FUNCTION "Gest Output" : VOID
TITLE =Gestione Output
AUTHOR : MassimoZ
FAMILY : NovaSrl
VERSION : 0.1

BEGIN
NETWORK
TITLE =R0 = Ripristino Emergenza
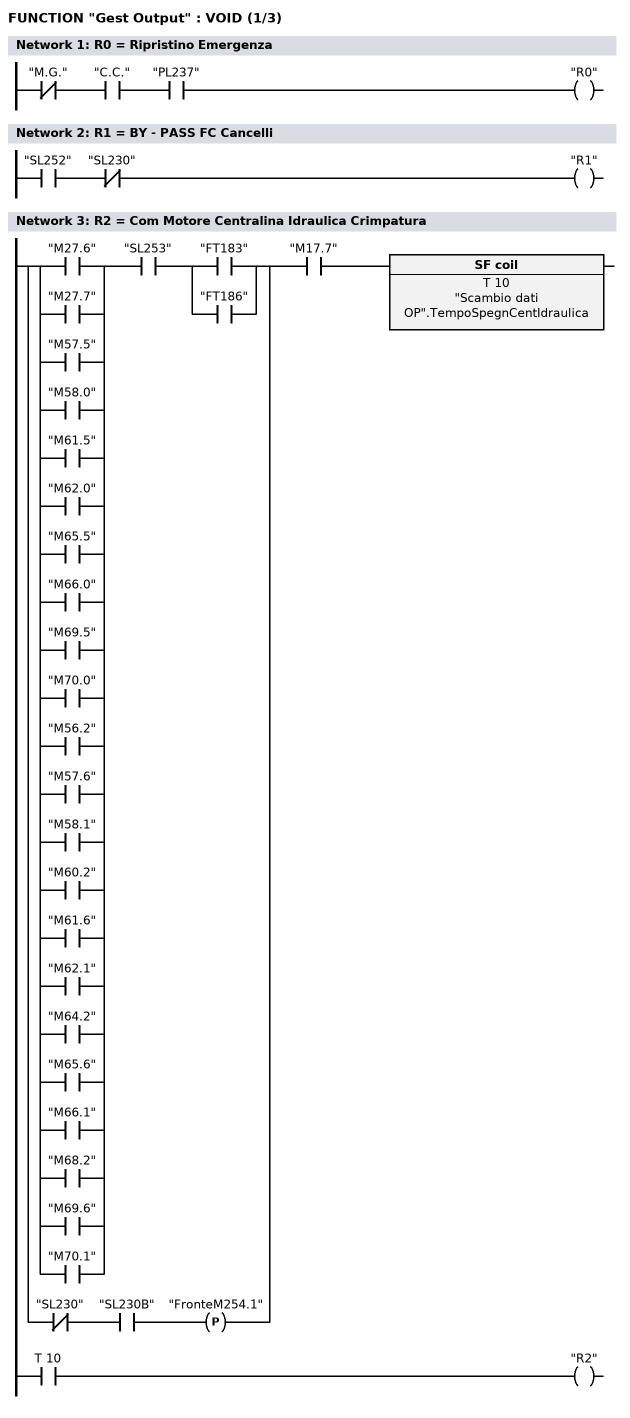
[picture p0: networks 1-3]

      UN    "M.G.";
      U     "C.C.";
      U     "PL237";
      =     "R0";
NETWORK
TITLE =R1 = BY - PASS FC Cancelli

      U     "SL252";
      UN    "SL230";
      =     "R1";

NETWORK
TITLE =R2 = Com Motore Centralina Idraulica Crimpatura

      U(    ;
      U(    ;
      O     "M27.6";

      O     "M27.7";
      O     "M57.5";
      O     "M58.0";
      O     "M61.5";
      O     "M62.0";
      O     "M65.5";
      O     "M66.0";
      O     "M69.5";
      O     "M70.0";
      O     "M56.2";
      O     "M57.6";
      O     "M58.1";
      O     "M60.2";
      O     "M61.6";
      O     "M62.1";
      O     "M64.2";
      O     "M65.6";
      O     "M66.1";
      O     "M68.2";
      O     "M69.6";
      O     "M70.1";
      )     ;
      U     "SL253";
      U(    ;
      O     "FT183";
      O     "FT186";
      )     ;
      O(    ;
      UN    "SL230";
      U     "SL230B";
      FP    "FronteM254.1";
      )     ;
      )     ;
      U     "M17.7";
      L     "Scambio dati OP".TempoSpegnCentIdraulica;
      SA    T     10;
      NOP   0;
      NOP   0;
      NOP   0;
      U     T     10;
      =     "R2";
NETWORK
TITLE =R3 = Com Start Motore Spazzole
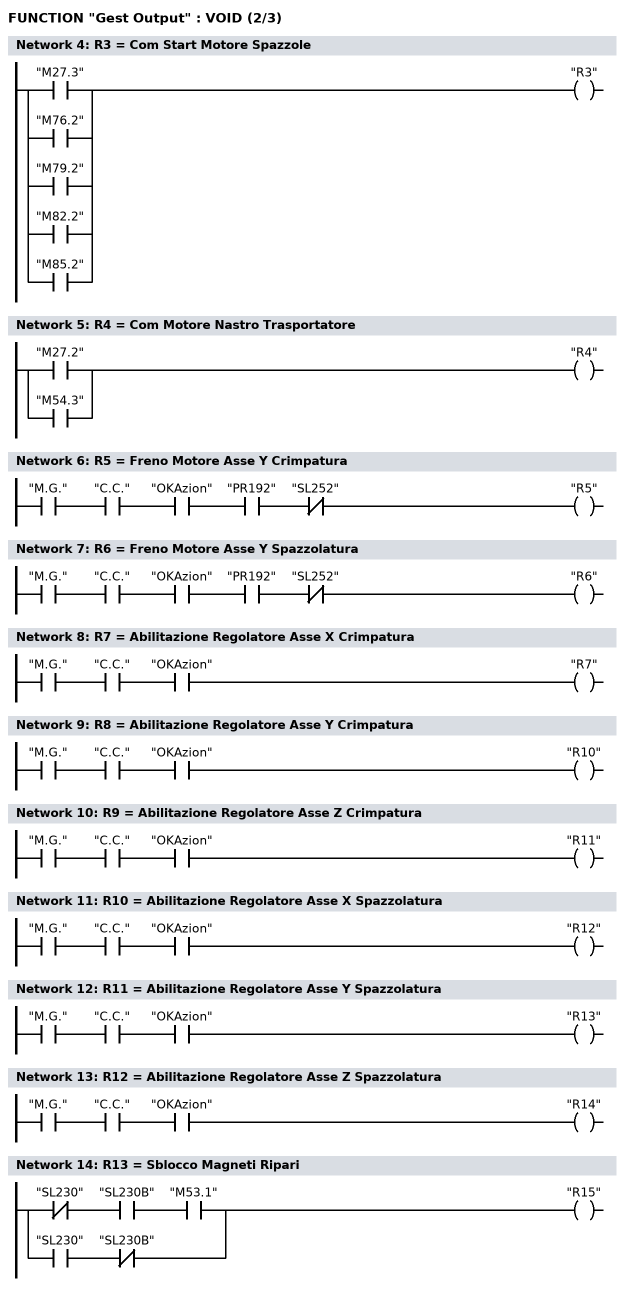
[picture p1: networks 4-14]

      O     "M27.3";
      O     "M76.2";

      O     "M79.2";
      O     "M82.2";
      O     "M85.2";
      =     "R3";
NETWORK
TITLE =R4 = Com Motore Nastro Trasportatore

      O     "M27.2";
      O     "M54.3";
      =     "R4";
NETWORK
TITLE =R5 = Freno Motore Asse Y Crimpatura

      U     "M.G.";
      U     "C.C.";
      U     "OKAzion";
      U     "PR192";
      UN    "SL252";
      =     "R5";
NETWORK
TITLE =R6 = Freno Motore Asse Y Spazzolatura

      U     "M.G.";
      U     "C.C.";
      U     "OKAzion";
      U     "PR192";
      UN    "SL252";
      =     "R6";
NETWORK
TITLE =R7 = Abilitazione Regolatore Asse X Crimpatura

      U     "M.G.";
      U     "C.C.";
      U     "OKAzion";
      =     "R7";
NETWORK
TITLE =R8 = Abilitazione Regolatore Asse Y Crimpatura

      U     "M.G.";
      U     "C.C.";
      U     "OKAzion";
      =     "R10";
NETWORK
TITLE =R9 = Abilitazione Regolatore Asse Z Crimpatura

      U     "M.G.";
      U     "C.C.";
      U     "OKAzion";
      =     "R11";
NETWORK
TITLE =R10 = Abilitazione Regolatore Asse X Spazzolatura

      U     "M.G.";
      U     "C.C.";
      U     "OKAzion";
      =     "R12";
NETWORK
TITLE =R11 = Abilitazione Regolatore Asse Y Spazzolatura

      U     "M.G.";
      U     "C.C.";
      U     "OKAzion";
      =     "R13";
NETWORK
TITLE =R12 = Abilitazione Regolatore Asse Z Spazzolatura

      U     "M.G.";
      U     "C.C.";
      U     "OKAzion";
      =     "R14";
NETWORK
TITLE =R13 = Sblocco Magneti Ripari

      UN    "SL230";
      U     "SL230B";
      U     "M53.1";
      O     ;
      U     "SL230";
      UN    "SL230B";
      =     "R15";
NETWORK
TITLE =Power On Reset Azionamenti (Reset Allarme Tensione Insufficente)
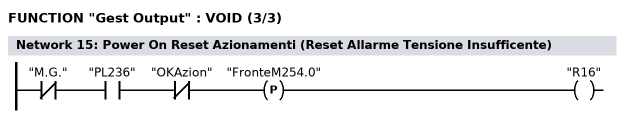
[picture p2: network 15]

      UN    "M.G.";
      U     "PL236";
      UN    "OKAzion";
      FP    "FronteM254.0";
      =     "R16";
NETWORK
TITLE =Scorta

      CLR   ;
      =     A      1.7;
NETWORK
TITLE =EV160 = Com Rotazione Polso a 45 gradi
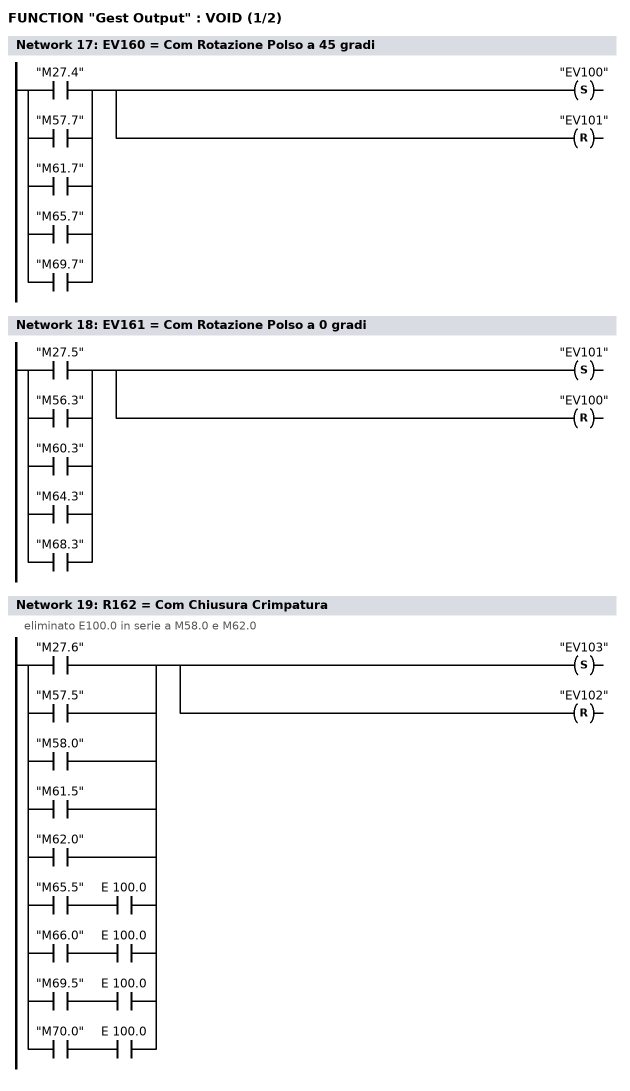
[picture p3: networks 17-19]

      O     "M27.4";
      O     "M57.7";
      O     "M61.7";
      O     "M65.7";
      O     "M69.7";
      S     "EV100";
      R     "EV101";
NETWORK
TITLE =EV161 = Com Rotazione Polso a 0 gradi

      O     "M27.5";
      O     "M56.3";
      O     "M60.3";
      O     "M64.3";
      O     "M68.3";
      S     "EV101";
      R     "EV100";
NETWORK
TITLE =R162 = Com Chiusura Crimpatura
//eliminato E100.0 in serie a M58.0 e M62.0
      O     "M27.6";
      O     "M57.5";
      O     "M58.0";
      O     "M61.5";
      O     "M62.0";
      O     ;
      U     "M65.5";
      U     E    100.0;
      O     ;
      U     "M66.0";
      U     E    100.0;
      O     ;
      U     "M69.5";
      U     E    100.0;
      O     ;
      U     "M70.0";
      U     E    100.0;
      S     "EV103";
      R     "EV102";
NETWORK
TITLE =R163 = Com Apertura Crimpatura
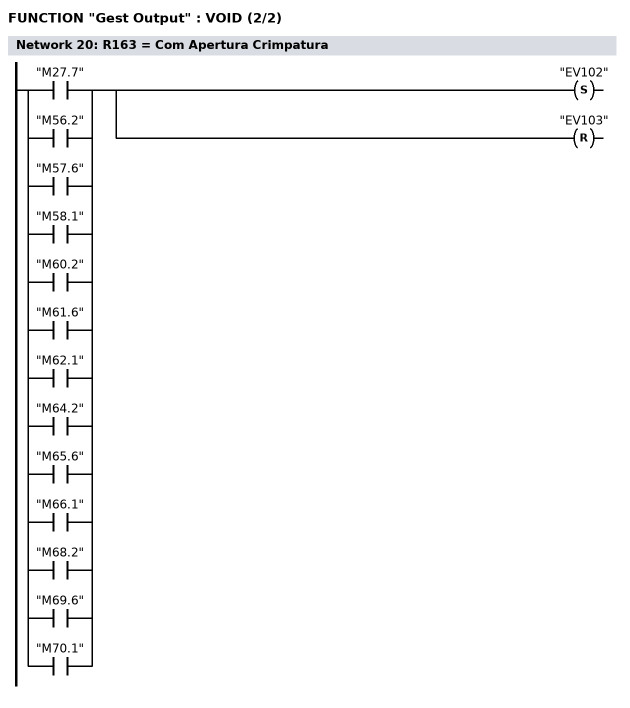
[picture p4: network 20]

      O     "M27.7";
      O     "M56.2";
      O     "M57.6";
      O     "M58.1";
      O     "M60.2";
      O     "M61.6";
      O     "M62.1";
      O     "M64.2";
      O     "M65.6";
      O     "M66.1";
      O     "M68.2";
      O     "M69.6";
      O     "M70.1";
      S     "EV102";
      R     "EV103";
NETWORK
TITLE =EV164 = Scorta

      CLR   ;
      =     A     16.0;
NETWORK
TITLE =EV165 = Scorta

      CLR   ;
      =     A     16.1;
NETWORK
TITLE =R166 = Com Avanti Cadenziatore in entrata
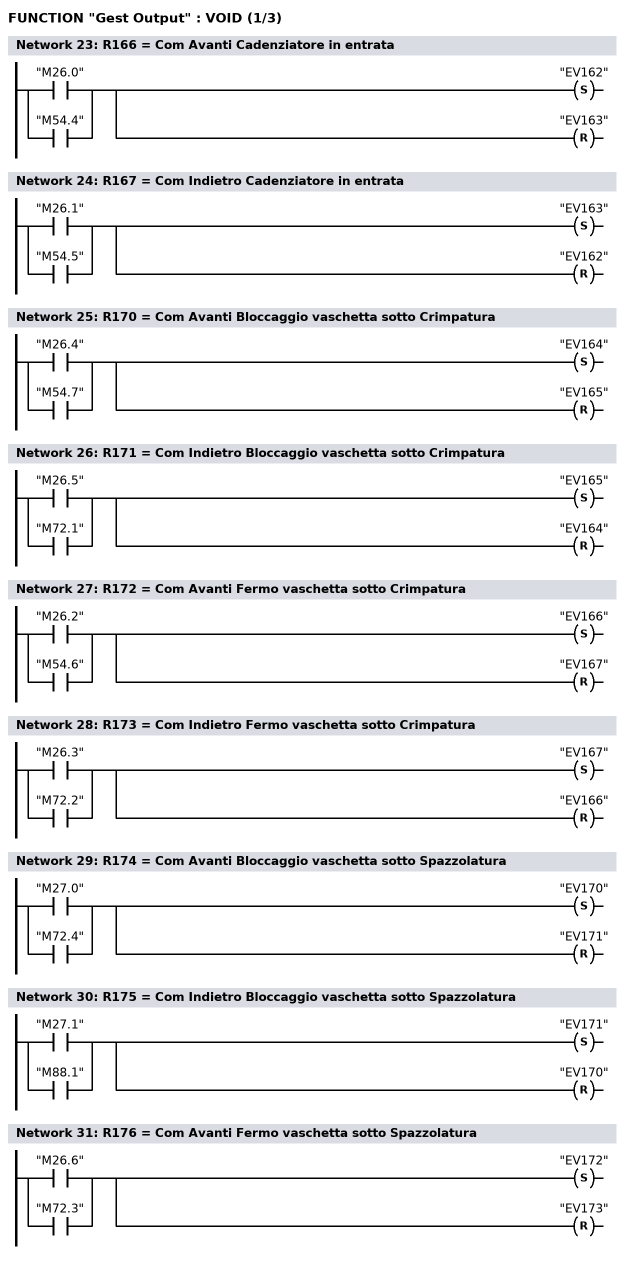
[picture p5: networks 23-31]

      O     "M26.0";
      O     "M54.4";
      S     "EV162";
      R     "EV163";
NETWORK
TITLE =R167 = Com Indietro Cadenziatore in entrata

      O     "M26.1";
      O     "M54.5";
      S     "EV163";
      R     "EV162";
NETWORK
TITLE =R170 = Com Avanti Bloccaggio vaschetta sotto Crimpatura

      O     "M26.4";
      O     "M54.7";
      S     "EV164";
      R     "EV165";
NETWORK
TITLE =R171 = Com Indietro Bloccaggio vaschetta sotto Crimpatura

      O     "M26.5";
      O     "M72.1";
      S     "EV165";
      R     "EV164";
NETWORK
TITLE =R172 = Com Avanti Fermo vaschetta sotto Crimpatura

      O     "M26.2";
      O     "M54.6";
      S     "EV166";
      R     "EV167";
NETWORK
TITLE =R173 = Com Indietro Fermo vaschetta sotto Crimpatura

      O     "M26.3";
      O     "M72.2";
      S     "EV167";
      R     "EV166";
NETWORK
TITLE =R174 = Com Avanti Bloccaggio vaschetta sotto Spazzolatura

      O     "M27.0";
      O     "M72.4";
      S     "EV170";
      R     "EV171";
NETWORK
TITLE =R175 = Com Indietro Bloccaggio vaschetta sotto Spazzolatura

      O     "M27.1";
      O     "M88.1";
      S     "EV171";
      R     "EV170";
NETWORK
TITLE =R176 = Com Avanti Fermo vaschetta sotto Spazzolatura

      O     "M26.6";
      O     "M72.3";
      S     "EV172";
      R     "EV173";
NETWORK
TITLE =R177 = Com Indietro Fermo vaschetta sotto Spazzolatura
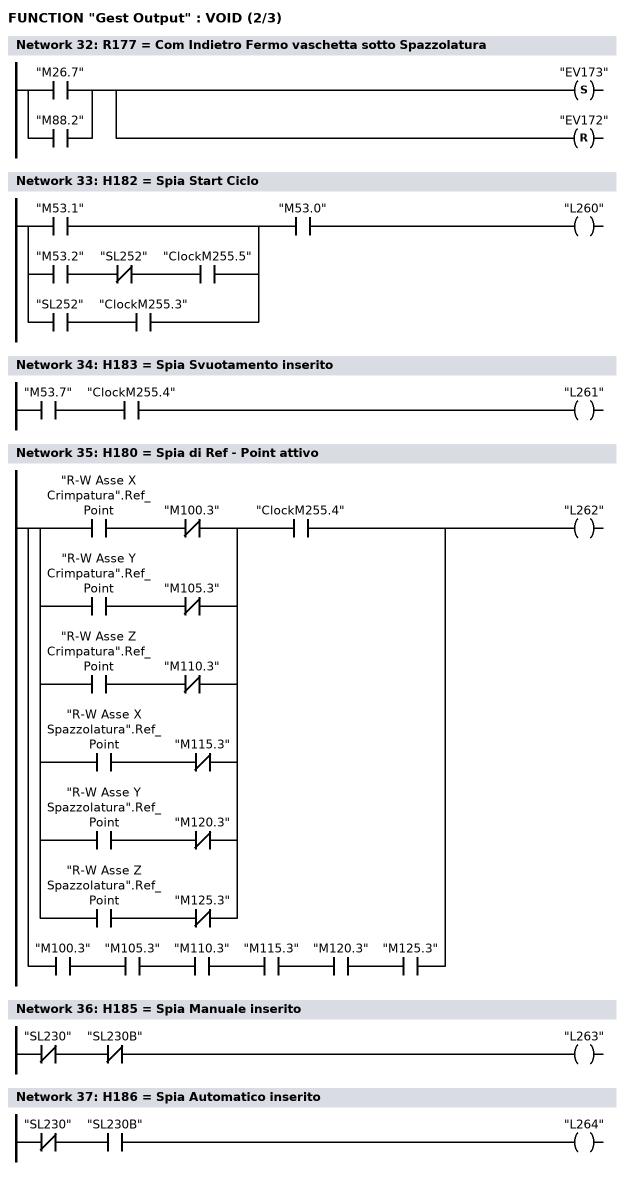
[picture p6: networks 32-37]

      O     "M26.7";
      O     "M88.2";
      S     "EV173";
      R     "EV172";
NETWORK
TITLE =H182 = Spia Start Ciclo

      U(    ;
      O     "M53.1";
      O     ;
      U     "M53.2";
      UN    "SL252";
      U     "ClockM255.5";
      O     ;
      U     "SL252";
      U     "ClockM255.3";
      )     ;
      U     "M53.0";
      =     "L260";
NETWORK
TITLE =H183 = Spia Svuotamento inserito

      U     "M53.7";
      U     "ClockM255.4";
      =     "L261";
NETWORK
TITLE =H180 = Spia di Ref - Point attivo

      U(    ;
      U     "R-W Asse X Crimpatura".Ref_Point;
      UN    "M100.3";
      O     ;
      U     "R-W Asse Y Crimpatura".Ref_Point;
      UN    "M105.3";
      O     ;
      U     "R-W Asse Z Crimpatura".Ref_Point;
      UN    "M110.3";
      O     ;
      U     "R-W Asse X Spazzolatura".Ref_Point;
      UN    "M115.3";
      O     ;
      U     "R-W Asse Y Spazzolatura".Ref_Point;
      UN    "M120.3";
      O     ;
      U     "R-W Asse Z Spazzolatura".Ref_Point;
      UN    "M125.3";
      )     ;
      U     "ClockM255.4";
      O     ;
      U     "M100.3";
      U     "M105.3";
      U     "M110.3";
      U     "M115.3";
      U     "M120.3";
      U     "M125.3";
      =     "L262";
NETWORK
TITLE =H185 = Spia Manuale inserito

      UN    "SL230";
      UN    "SL230B";
      =     "L263";
NETWORK
TITLE =H186 = Spia Automatico inserito

      UN    "SL230";
      U     "SL230B";
      =     "L264";
NETWORK
TITLE =H184 = Spia Presenza Allarme
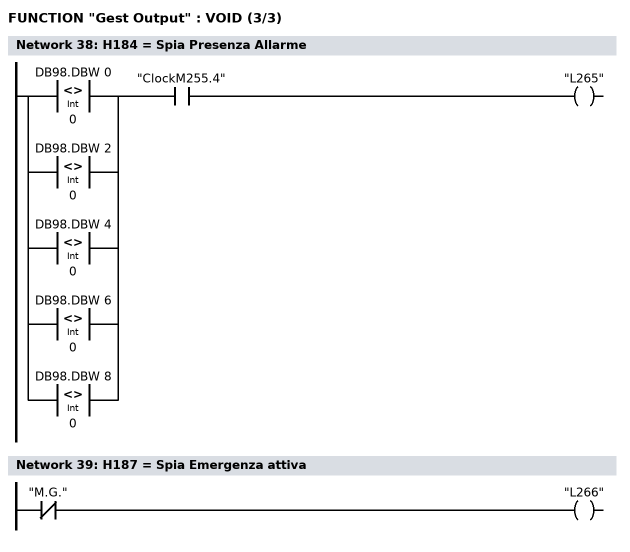
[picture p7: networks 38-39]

      U(    ;
      O(    ;
      L     DB98.DBW    0;
      L     0;
      <>I   ;
      )     ;
      O(    ;
      L     DB98.DBW    2;
      L     0;
      <>I   ;
      )     ;
      O(    ;
      L     DB98.DBW    4;
      L     0;
      <>I   ;
      )     ;
      O(    ;
      L     DB98.DBW    6;
      L     0;
      <>I   ;
      )     ;
      O(    ;
      L     DB98.DBW    8;
      L     0;
      <>I   ;
      )     ;
      )     ;
      U     "ClockM255.4";
      =     "L265";
NETWORK
TITLE =H187 = Spia Emergenza attiva

      UN    "M.G.";
      =     "L266";
NETWORK
TITLE =Scorta

      CLR   ;
      =     "A26.7";
NETWORK
TITLE =Jog + Attivo Pulsantiera Mobile
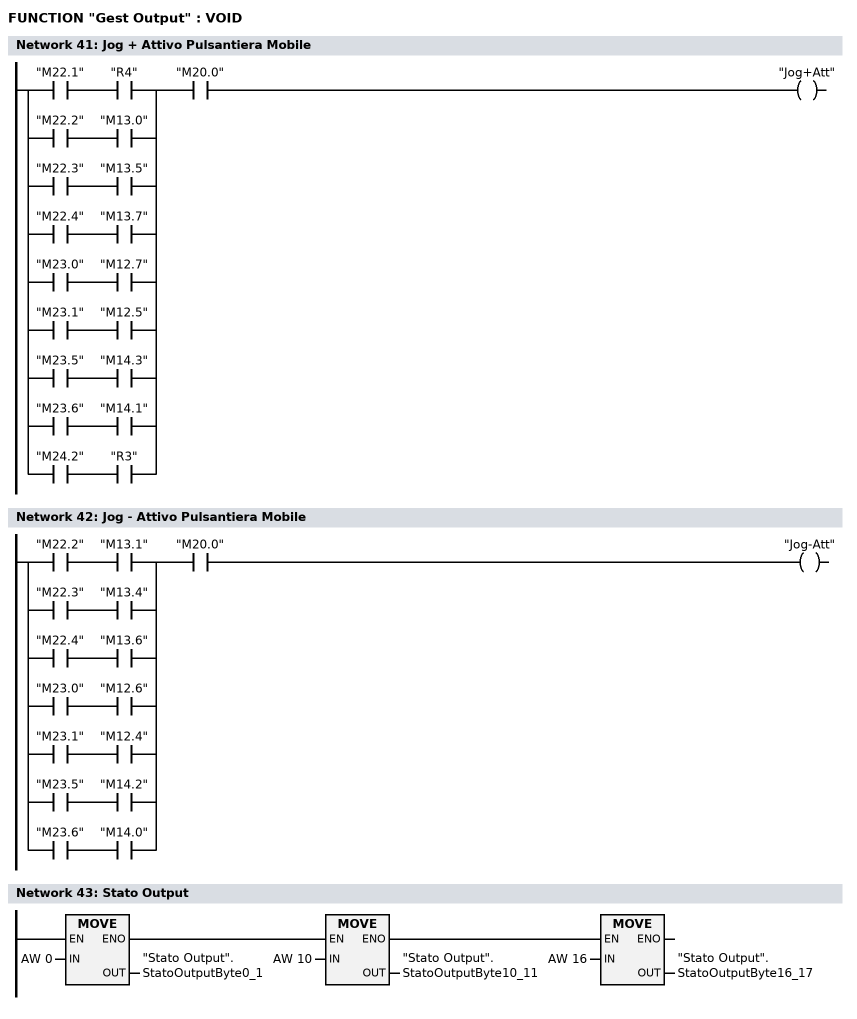
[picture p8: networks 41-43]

      U(    ;
      U     "M22.1";
      U     "R4";
      O     ;
      U     "M22.2";
      U     "M13.0";
      O     ;
      U     "M22.3";
      U     "M13.5";
      O     ;
      U     "M22.4";
      U     "M13.7";
      O     ;
      U     "M23.0";
      U     "M12.7";
      O     ;
      U     "M23.1";
      U     "M12.5";
      O     ;
      U     "M23.5";
      U     "M14.3";
      O     ;
      U     "M23.6";
      U     "M14.1";
      O     ;
      U     "M24.2";
      U     "R3";
      )     ;
      U     "M20.0";
      =     "Jog+Att";
NETWORK
TITLE =Jog - Attivo Pulsantiera Mobile

      U(    ;
      U     "M22.2";
      U     "M13.1";
      O     ;
      U     "M22.3";
      U     "M13.4";
      O     ;
      U     "M22.4";
      U     "M13.6";
      O     ;
      U     "M23.0";
      U     "M12.6";
      O     ;
      U     "M23.1";
      U     "M12.4";
      O     ;
      U     "M23.5";
      U     "M14.2";
      O     ;
      U     "M23.6";
      U     "M14.0";
      )     ;
      U     "M20.0";
      =     "Jog-Att";
NETWORK
TITLE =Stato Output

      U(    ;
      U(    ;
      L     AW     0;
      T     "Stato Output".StatoOutputByte0_1;
      SET   ;
      SAVE  ;
      CLR   ;
      U     BIE;
      )     ;
      SPBNB _001;
      L     AW    10;
      T     "Stato Output".StatoOutputByte10_11;
      SET   ;
      SAVE  ;
      CLR   ;
_001: U     BIE;
      )     ;
      SPBNB _002;
      L     AW    16;
      T     "Stato Output".StatoOutputByte16_17;
_002: NOP   0;
END_FUNCTION

